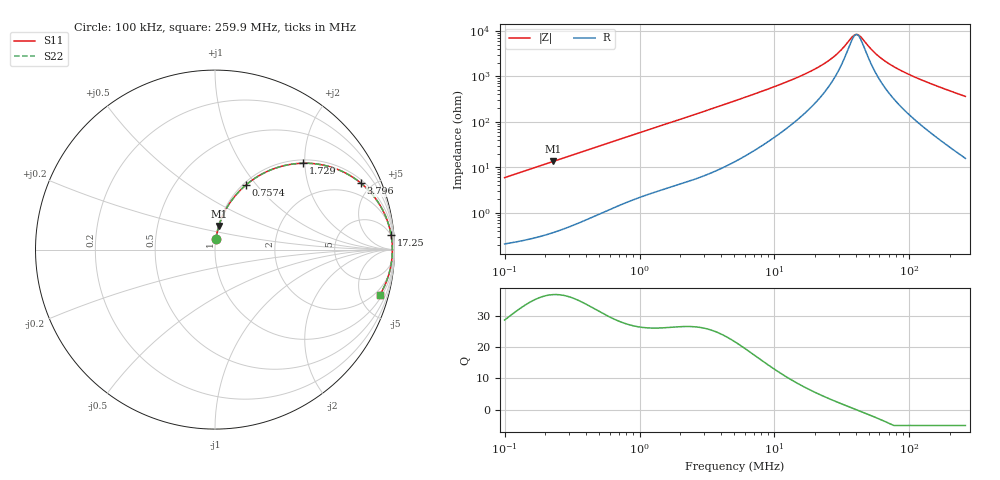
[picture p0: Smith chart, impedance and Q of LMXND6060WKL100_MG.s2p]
! LMXND6060WKL100_MG  S-PARAMETER MODEL  ( General Type )
! Model Generated by TAIYO YUDEN Corporation (http://www.ty-top.com)
! Version 1.0
! TAIYO YUDEN Control No. 191025NI43SB-FBB
! Copyright(c) 2019 TAIYO YUDEN CO.,LTD. All Rights Reserved.
! Product Description (link to TY-COMPAS)
! https://ds.yuden.co.jp/TYCOMPAS/or/detail?pn=LMXND6060WKL100MMG&u=M
! Products Name : Inductors
! Characteristics :
!  Inductance : 10 uH , SRF(min) : 18 MHz , DC Resistance(max) : 0.15 Ohm
!  Rated Current : Saturation :1900 mA , Temp Rise : 1500 mA
!  Case Size : 6.0 x 6.0 / 0.236 x 0.236 [mm/inch] , Thickness : 2 / 0.079 [mm/inch]
!  (Conditions: Temperature = 25 degC , DC Bias Current/Voltage = 0A / 0V)
! External Node Assignments :
!  1  o---GGG---o  2
! GND o---------o GND
! Frequency Range : 0.1MHz  -  259.929867MHz  [ 402 STEP ]
# MHz S RI R 50
! Freq[MHz].  S11 Real  S11 Imag  S21 Real  S21 Imag  S12 Real  S12 Imag  S22 Real  S22 Imag
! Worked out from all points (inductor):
!   401 points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, 100 kHz to 259.9 MHz, reference 50 ohm
!   read as one part in series: L = 9.44 uH near 104 kHz
!   highest Q = 36.7 at 228.3 kHz (marker M1), where L = 9.41 uH
!   self-resonance near 40.16 MHz
!   S11 on the Smith chart (normalised r, x): 100 kHz: 1.00, +0.12; 757.4 kHz: 1.03, +0.88; 1.729 MHz: 1.07, +1.97; 3.796 MHz: 1.17, +4.30; 17.25 MHz: 4, +23; 259.9 MHz: 1.32, -7.24
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0.1  0.00557 0.059  0.9944 -0.059  0.9944 -0.059  0.00557 0.059
0.228328  0.0213 0.1316  0.9787 -0.1316  0.9787 -0.1316  0.0213 0.1316
0.37324  0.0515 0.2069  0.9485 -0.2069  0.9485 -0.2069  0.0515 0.2069
0.7574  0.1708 0.3587  0.8292 -0.3587  0.8292 -0.3587  0.1708 0.3587
1.393082  0.392 0.4694  0.608 -0.4694  0.608 -0.4694  0.392 0.4694
1.72936  0.4922 0.4813  0.5078 -0.4813  0.5078 -0.4813  0.4922 0.4813
2.463508  0.6551 0.4569  0.3449 -0.4569  0.3449 -0.4569  0.6551 0.4569
3.796391  0.8126 0.3705  0.1874 -0.3705  0.1874 -0.3705  0.8126 0.3705
5.098332  0.8831 0.299  0.1169 -0.299  0.1169 -0.299  0.8831 0.299
10.14444  0.9617 0.1566  0.0383 -0.1566  0.0383 -0.1566  0.9617 0.1566
17.24769  0.981 0.0822  0.019 -0.0822  0.019 -0.0822  0.981 0.0822
19.02902  0.9828 0.071  0.0172 -0.071  0.0172 -0.071  0.9828 0.071
23.16263  0.9855 0.0506  0.0145 -0.0506  0.0145 -0.0506  0.9855 0.0506
27.64535  0.987 0.0337  0.013 -0.0337  0.013 -0.0337  0.987 0.0337
31.72358  0.9877 0.0213  0.0123 -0.0213  0.0123 -0.0213  0.9877 0.0213
37.86312  0.9881 0.00587  0.0119 -0.00587  0.0119 -0.00587  0.9881 0.00587
40.16316  0.9882 0.000791  0.0118 -0.000791  0.0118 -0.000791  0.9882 0.000791
43.44866  0.9881 -0.00598  0.0119 0.00598  0.0119 0.00598  0.9881 -0.00598
56.09953  0.9874 -0.0284  0.0126 0.0284  0.0126 0.0284  0.9874 -0.0284
71.02397  0.9856 -0.0507  0.0144 0.0507  0.0144 0.0507  0.9856 -0.0507
118.4051  0.9759 -0.1096  0.0241 0.1096  0.0241 0.1096  0.9759 -0.1096
259.9299  0.9199 -0.2506  0.0801 0.2506  0.0801 0.2506  0.9199 -0.2506
